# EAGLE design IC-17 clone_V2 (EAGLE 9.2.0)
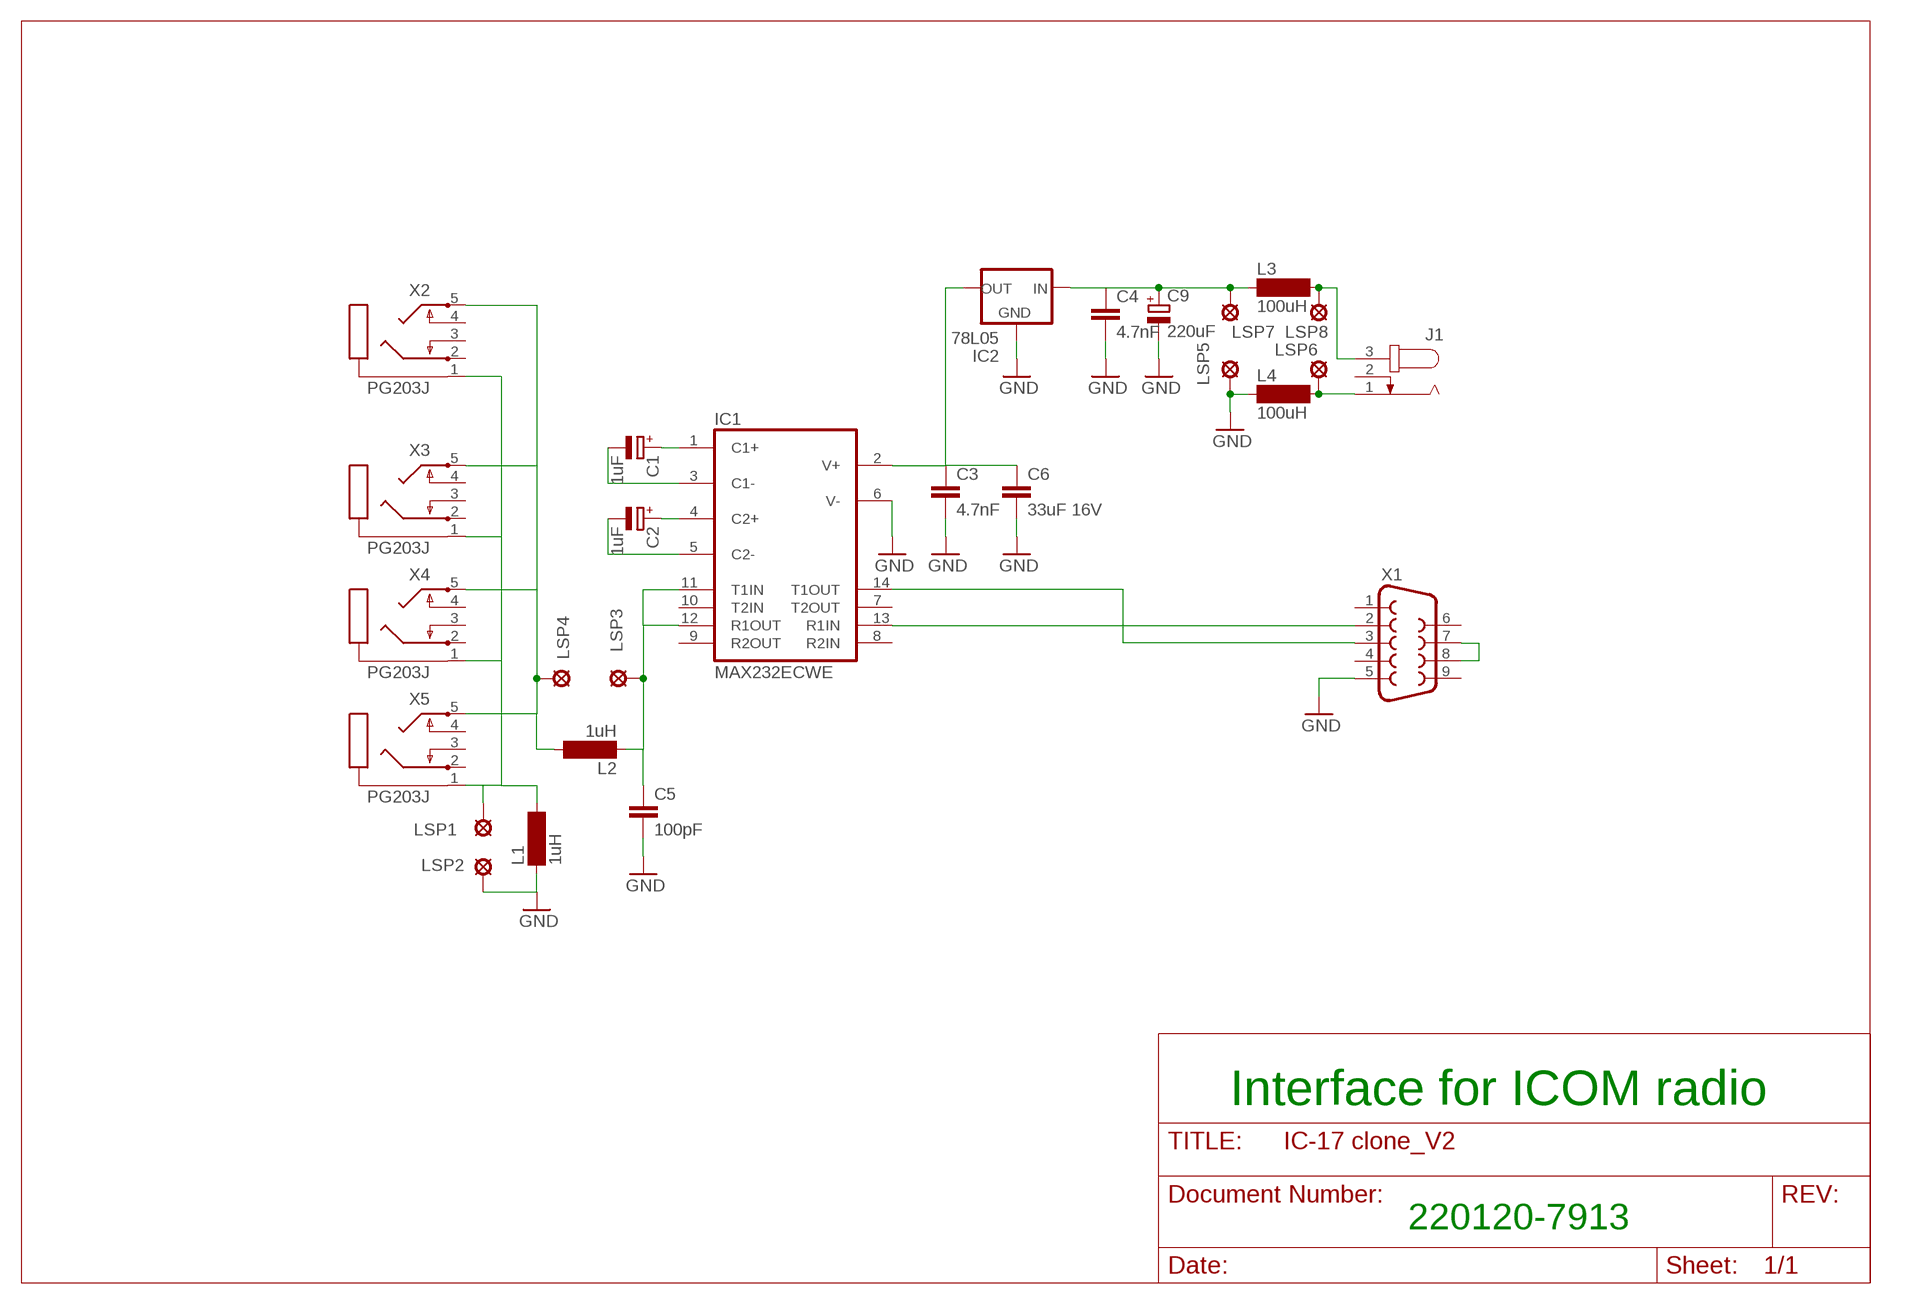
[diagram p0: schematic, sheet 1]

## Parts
C1  1uF  CPOL-EUSMCB  [SMC_B]
C2  1uF  CPOL-EUSMCB  [SMC_B]
C3  4.7nF  C-EUC0805K  [C0805K]
C4  4.7nF  C-EUC0805K  [C0805K]
C5  100pF  C-EUC0805  [C0805]
C6  33uF 16V  C-EUC1808  [C1808]
C9  220uF  CPOL-EUE5-8.5  [E5-8,5]
IC1  MAX232ECWE  [SO16L]
IC2  78L05  79LXX  [79LXX]
J1  JACK-PLUG0  [SPC4077]
L1  1uH  SM-1206  [SM-1206]
L2  1uH  SM-1206  [SM-1206]
L3  100uH  SM-1206  [SM-1206]
L4  100uH  SM-1206  [SM-1206]
LSP1  MCS08  [MCS08]
LSP2  MCS08  [MCS08]
LSP3  MCS08  [MCS08]
LSP4  MCS08  [MCS08]
LSP5  MCS08  [MCS08]
LSP6  MCS08  [MCS08]
LSP7  MCS08  [MCS08]
LSP8  MCS08  [MCS08]
X1  F09HP  [F09HP]
X2  PG203J  [PG203J]
X3  PG203J  [PG203J]
X4  PG203J  [PG203J]
X5  PG203J  [PG203J]

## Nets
GND: C3.2 C4.2 C5.2 C6.2 C9.- IC1.6(V-) IC2.GND L1.1 L4.1 LSP2.MP LSP5.MP X1.5
N$1: L1.2 LSP1.MP X2.1 X5.1
N$2: L2.2 LSP4.MP X2.5 X3.5 X4.5 X5.5
N$3: X3.1
N$4: X4.1
N$5: C1.+ IC1.1(C1+)
N$6: C1.- IC1.3(C1-)
N$7: C2.+ IC1.4(C2+)
N$8: C2.- IC1.5(C2-)
N$9: C5.1 IC1.11(T1IN) IC1.12(R1OUT) L2.1 LSP3.MP
N$10: IC1.14(T1OUT) X1.3
N$12: IC1.13(R1IN) X1.2
N$13: C3.1 C6.1 IC1.2(V+) IC2.OUT
N$14: C4.1 C9.+ IC2.IN L3.1 LSP7.MP
N$15: J1.3 L3.2 LSP8.MP
N$16: J1.1 L4.2 LSP6.MP
N$17: X1.7 X1.8
Unconnected: IC1.7(T2OUT) IC1.8(R2IN) IC1.9(R2OUT) IC1.10(T2IN) J1.2 X1.1 X1.4 X1.6 X1.9 X2.2 X2.3 X2.4 X3.2 X3.3 X3.4 X4.2 X4.3 X4.4 X5.2 X5.3 X5.4

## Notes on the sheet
- Interface for ICOM radio
- 220120-7913

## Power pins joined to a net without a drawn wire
GND: IC1.15(GND)
VCC: IC1.16(VCC)

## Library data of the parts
C1 C2 C9 = rcl:CPOL-EU: POLARIZED CAPACITOR, European symbol; SPICEPREFIX: C
C3-C6 = resistor:C-EU: CAPACITOR, European symbol
IC1 = maxim:MAX232ECWE: RS232 TRANSCEIVER; MF: MAXIM; MPN: MAX232ECWE+; OC_FARNELL: 9724435; OC_NEWARK: 67K4440
IC2 = v-reg:79LXX: VOLTAGE REGULATOR
J1 = con-jack:JACK-PLUG: DC POWER JACK Power Jack, DC, Right Angle, Through Hole, Rated 5A at 16VDC, PC Terminals Distributor: Farnell (www.Farnell.de) Drawing: 84N1161.pdf / 84N1162.pdf Manufacturer: SPC Technology (www.spctechnology.com) Type: SPC4077 / SPC 4078; OC_FARNELL: unknown; OC_NEWARK: unknown
L1-L4 = inductor-neosid:SM-1206: INDUCTOR; OC_FARNELL: unknown; OC_NEWARK: unknown
LSP1-LSP8 = solpad:MCS08: SOLDER PAD
X1 = con-subd:F09: SUB-D; OC_FARNELL: unknown; OC_NEWARK: unknown
X2-X5 = con-hirschmann:PG203J: MIC/HEADPHONE JACK KS-S stereo microphone/headphone jack PG203JN (Schukat); OC_FARNELL: unknown; OC_NEWARK: unknown

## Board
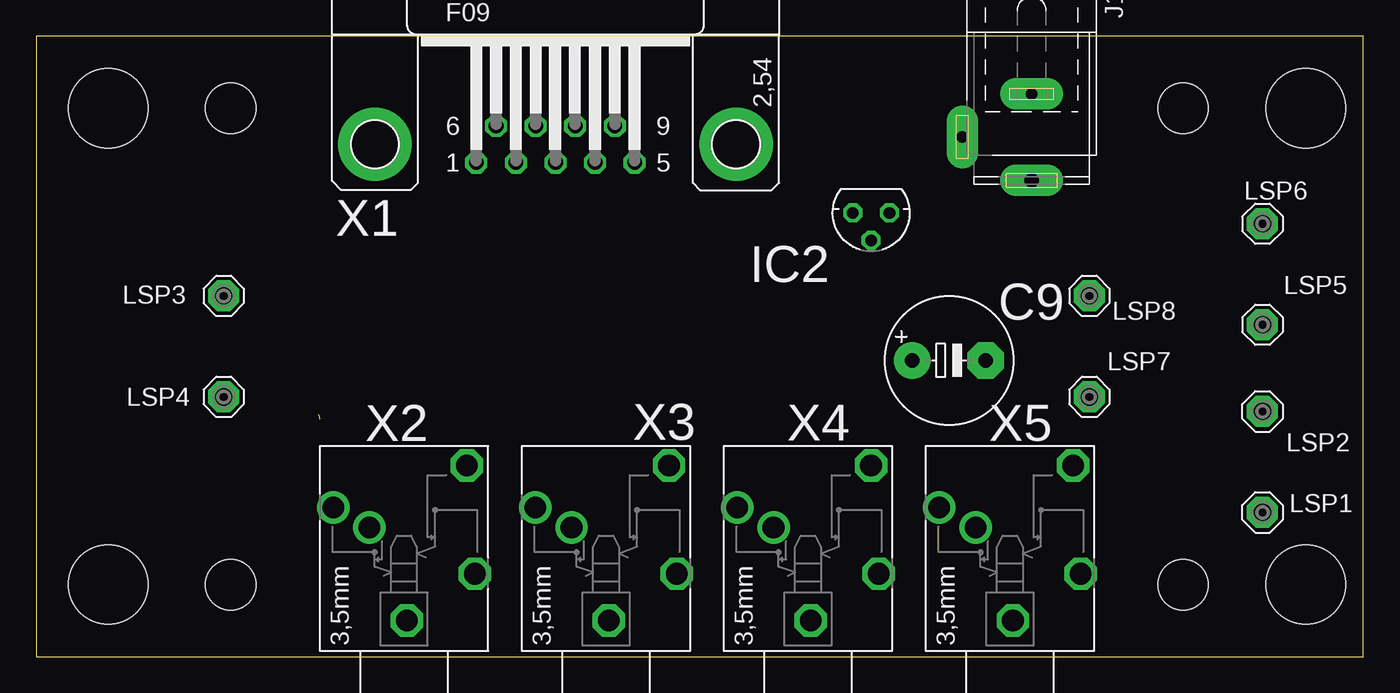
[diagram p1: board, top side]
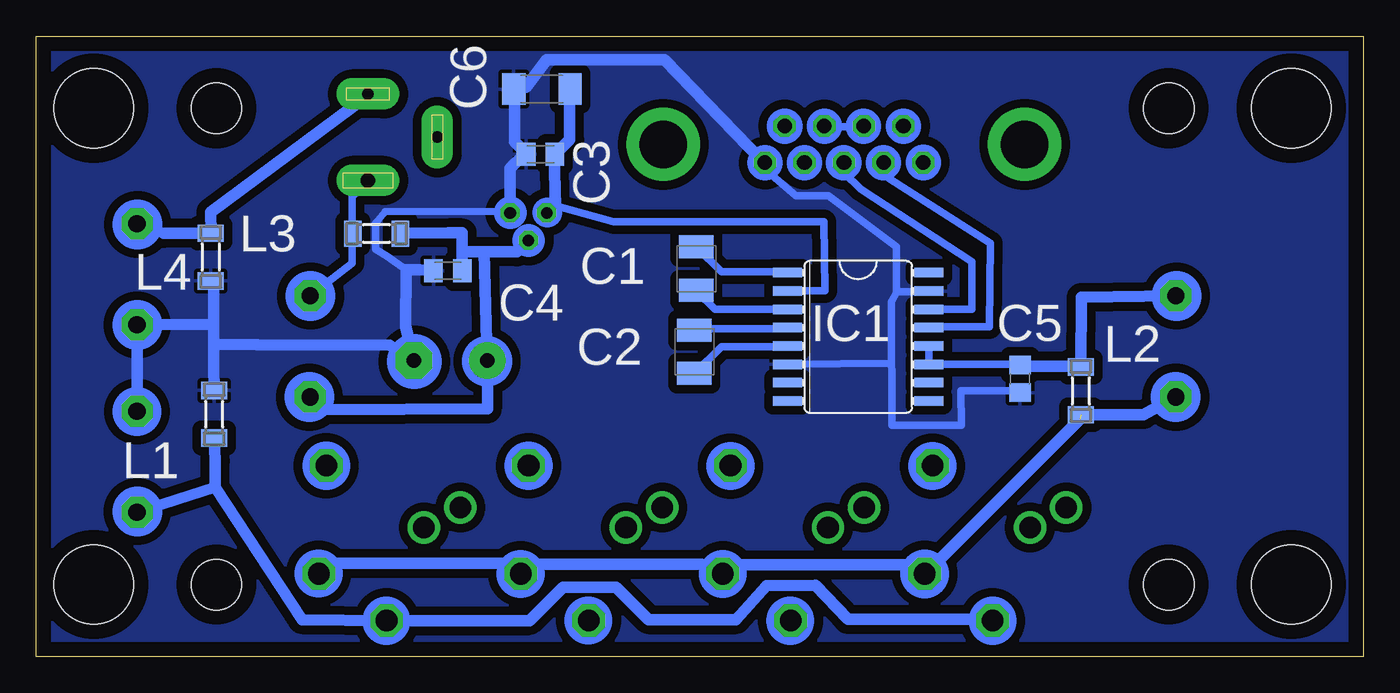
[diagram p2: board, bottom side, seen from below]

Size 92 x 43 mm. Coordinates in mm from the lower left corner, seen from the top.
Outline: 0,0 92,0 92,43 0,43 0,0
Copper layers (1*16): Top 0.035mm / dielectric 1.5mm / Bottom 0.035mm
Design rules "default": minimum track width 6mil, minimum drill 0.35mm, track to track 6mil, track to pad 6mil, pad to pad 6mil, via to via 6mil, smd to smd 6mil, copper to edge 40mil, drill to drill 6mil, minimum pad ring 10mil, minimum via ring 8mil, stop-mask expansion 4mil, vias tented up to drill 0mil, thermal gap 10mil
Holes 5.5 mm at 5,38 5,5 88,38 88,5
Holes 3.5 mm at 13.5,38 79.5,38 79.5,5 13.5,5

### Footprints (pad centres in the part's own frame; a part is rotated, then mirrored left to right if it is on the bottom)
SMC_B = smd 1.6 x 2.4: + -1.5,0; - 1.5,0
C0805K = smd 1.3 x 1.6: 1 -1,0; 2 1,0
C0805 = smd 1.3 x 1.5: 1 -0.95,0; 2 0.95,0
C1808 = smd 1.6 x 2.2: 1 -1.95,0; 2 1.95,0
E5-8,5 = drill 1.016 pad 2.54: + -2.54,0 | drill 1.016 pad 2.54 octagon: - 2.54,0
SO16L = smd 0.66 x 2.032: 1 -4.445,-4.902; 2 -3.175,-4.902; 3 -1.905,-4.902; 4 -0.635,-4.902; 5 0.635,-4.902; 6 1.905,-4.902; 7 3.175,-4.902; 8 4.445,-4.902; 9 4.445,4.902; 10 3.175,4.902; 11 1.905,4.902; 12 0.635,4.902; 13 -0.635,4.902; 14 -1.905,4.902; 15 -3.175,4.902; 16 -4.445,4.902
79LXX = drill 0.813 octagon: GND -1.27,0; IN 0,1.905; OUT 1.27,0
SPC4077 = drill 0.8 pad 2.184 long: 1 -3,0; 2 0,-4.8 | drill 1 pad 2.184 long: 3 3,0
SM-1206 = smd 1.2 x 1.8: 1 -1.65,0; 2 1.65,0
MCS08 = drill 1.194 pad 2.159 octagon: MP 0,0
F09HP = drill 1.016 octagon: 1 -5.486,-1.27; 2 -2.743,-1.27; 3 0,-1.27; 4 2.743,-1.27; 5 5.486,-1.27; 6 -4.115,1.27; 7 -1.372,1.27; 8 1.372,1.27; 9 4.115,1.27 | drill 3.302 pad 5.08: G1 -12.522,0; G2 12.522,0
PG203J = drill 1.499 octagon: 1 -5.004,-0.203; 4 5.74,-4.369; 5 -1.753,-4.902 | drill 1.499: 2 2.845,4.902; 3 1.448,2.388

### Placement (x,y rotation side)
C1  46.24,26.89 270 bottom
C2  46.38,21.13 270 bottom
C3  57.04,34.81 180 bottom
C4  63.46,26.75 180 bottom
C5  23.8,19.25 270 bottom
C6  56.94,39.33 180 bottom
C9  63.27,20.52 0 top
IC1  35.02,22.16 270 bottom
IC2  57.88,30.75 180 top
J1  69,36 270 top
L1  79.65,16.8 270 bottom
L2  19.59,18.41 270 bottom
L3  68.4,29.32 180 bottom
L4  79.89,27.69 90 bottom
LSP1  85,10 90 top
LSP2  85,17 90 top
LSP3  13,25 0 top
LSP4  13,18 0 top
LSP5  85,23 0 top
LSP6  85,30 0 top
LSP7  73,18 0 top
LSP8  73,25 0 top
X1  36,35.5 0 top
X2  25.5,7.5 90 top
X3  39.5,7.5 90 top
X4  53.5,7.5 90 top
X5  67.5,7.5 90 top

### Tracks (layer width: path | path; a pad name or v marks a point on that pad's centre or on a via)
GND
  Top 0.152: 41.6,34.14 X1.5
  Bottom 0.152: 58.83,39.32 C6.2 58.67,39.47 | 58.06,34.9 C3.2 58.22,34.75 | 79.7,25.76 79.86,25.91 L4.1 | 30.63,25.3 30.18,25.3 IC1.15 | 23.93,18.44 C5.2 | 39.78,20.27 IC1.6
  Bottom 0.508: 66.34,26.8 67.67,27.74 68.45,28.22 68.45,30.05 67.79,30.84 59.99,30.86 IC2.GND 59.13,30.79 | 23.93,18.44 27.89,18.44 27.86,16.05 32.66,16.05 32.69,19.66 32.72,20.32 | 32.72,20.32 32.72,24.59 32.33,25.3 | 30.63,25.3 32.33,25.3 | 32.33,25.3 32.35,25.3 32.37,28.22 32.37,28.4 37.07,31.94 39.33,31.95 41.49,33.77 X1.5 41.6,34.29 | 32.72,20.32 39.78,20.27
  Bottom 0.813: 58.83,39.32 58.83,35.66 58.06,34.9 | 79.7,25.76 79.7,23.04 | 79.7,23.04 79.7,21.64 | 79.7,21.64 79.7,20.12 L1.1 | C4.2 65.43,26.8 66.34,26.8 66.37,22.86 C9.- 67.51,21.59 76.68,21.63 79.7,21.64 | 59.13,30.79 59.13,33.83 58.22,34.75 | 58.67,39.47 58.04,39.47 56.63,41.35 48.43,41.35 41.6,34.29 | LSP2.MP LSP5.MP 79.7,23.04
  pour Bottom (isolate 0.6): 0,43 92,43 92,0 0,0
N$1
  Bottom 0.152: 25.76,2.59 X2.1
  Bottom 0.508: 79.58,13.56 79.58,13.66
  Bottom 0.813: 79.58,11.73 79.58,13.56 L1.2 | 79.58,11.73 73.56,2.56 X5.1 57.8,2.5 55.47,4.83 51.82,4.83 49.55,2.56 43.48,2.56 41.36,4.91 37.97,4.94 35.74,2.59 25.76,2.59 | LSP1.MP 79.58,11.73
N$2  (1 unrouted)
  Top 0.152: 58.37,5.79 X4.5 58.52,5.79 | 44.5,5.79 X3.5 | 72.39,5.79 X5.5
  Bottom 0.152: 30.33,5.79 X2.5
  Bottom 0.508: 43.63,6.38 X3.5 45.87,6.4 | 31.52,6.38 X2.5 | 57.91,6.4 X4.5 59.14,6.48 | 71.67,6.48 X5.5
  Bottom 0.813: 30.33,5.79 19.66,16.46 | 43.63,6.38 31.52,6.38 | 57.91,6.4 45.87,6.4 | 71.67,6.48 59.14,6.48 | LSP4.MP 15.24,16.76 L2.2
N$5
  Bottom 0.152: 39.93,26.67 IC1.1 | 46.18,28.35 C1.+
  Bottom 0.508: 39.93,26.67 44.5,26.67 46.18,28.35
N$6
  Bottom 0.152: 46.18,25.3 C1.-
  Bottom 0.508: 46.18,25.3 44.96,24.08 IC1.3
N$7
  Bottom 0.152: 46.33,22.71 C2.+
  Bottom 0.508: 46.33,22.71 39.93,22.71 IC1.4
N$8
  Bottom 0.152: 39.93,21.49 IC1.5 | 46.33,19.66 C2.-
  Bottom 0.508: 39.93,21.49 44.5,21.49 46.33,19.66
N$9
  Bottom 0.152: 23.77,20.12 C5.1 | 19.66,20.12 L2.1 | 29.87,20.27 IC1.11
  Bottom 0.508: IC1.11 IC1.12 | 29.87,20.27 23.93,20.27 C5.1
  Bottom 0.813: 19.66,20.12 23.77,20.12 | L2.1 19.56,24.89 LSP3.MP
N$10
  Bottom 0.152: 30.63,24.08 30.18,24.08 IC1.14
  Bottom 0.508: 30.18,24.08 27.15,24.08 27.15,27.36 34.83,32.37 36,33.54 X1.3
N$12
  Bottom 0.152: 30.02,22.86 IC1.13 | 32.85,33.12 X1.2
  Bottom 0.508: 30.02,22.86 25.91,22.86 25.86,28.64 32.85,33.12
N$13
  Bottom 0.152: 56.54,30.79 IC2.OUT | 55.02,39.32 C6.1 | 55.93,34.9 C3.1
  Bottom 0.508: 56.54,30.79 55.98,31.24 51.97,30.12 37.39,30.12 37.34,25.35 39.37,25.35 IC1.2 | 56.08,34.75 C3.1
  Bottom 0.813: 55.98,31.24 56.08,34.75 | 55.02,39.32 55.02,35.81 55.93,34.9
N$14
  Bottom 0.152: 57.91,28.8 IC2.IN | 66.7,29.34 L3.1 | LSP7.MP 72.11,17.11 | 60.71,20.5 C9.+
  Bottom 0.508: 57.91,28.8 58.67,28.04 | 62.48,28.04 C4.1
  Bottom 0.813: 58.67,28.04 60.96,28.04 | 60.96,28.04 62.48,28.04 | 66.7,29.34 63.4,29.36 62.46,29.36 C4.1 | 60.96,28.04 C9.+ | 72.11,17.11 60.71,17.17 60.71,20.5
N$15
  Bottom 0.152: 70.1,28.96 L3.2 | 69.04,32.92 J1.3
  Bottom 0.508: 69.04,32.92 70.1,31.85 70.1,28.96 70.1,27.25 LSP8.MP
N$16
  Bottom 0.152: 79.86,29.41 L4.2 | 83.16,29.34 LSP6.MP
  Bottom 0.508: 69.04,38.86 J1.1
  Bottom 0.813: 79.86,29.41 79.88,30.81 69.04,38.86 | L4.2 83.16,29.34
N$17
  Bottom 0.152: 34.75,36.73 X1.7 | 37.34,36.73 X1.8
  Bottom 0.508: 37.34,36.73 34.75,36.73
(copper drawn outside any net)
  shapes: Bottom circle x34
